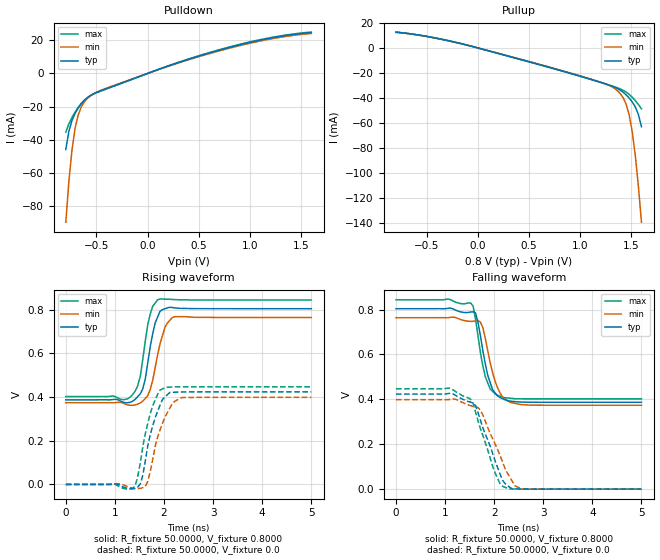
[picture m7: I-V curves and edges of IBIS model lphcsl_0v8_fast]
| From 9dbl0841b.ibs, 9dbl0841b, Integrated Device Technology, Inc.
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|   Model lphcsl_0v8_fast
[Model]  lphcsl_0v8_fast
Model_type Output
Polarity   Non-Inverting
Vmeas =  0.4000V
Cref =   2.0000pF
Rref =   0.0
Vref =   0.4000V
C_comp   1.1000pF   1.0000pF   1.2000pF
[Temperature Range]   27.0000   70.0000   0.0
[Voltage Range]   0.8000V   0.7600V   0.8400V
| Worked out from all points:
|   slope of the pulldown table from 0 to 0.12 V, typ, clamps not added: 44.4 ohm
|   slope of the pullup table from 0 to 0.12 V, typ, clamps not added: 45.4 ohm
|   rising waveform, R_fixture 50.0000, V_fixture 0.8000: 20-80 % time 197ps typ, 236ps min, 183ps max; typ from 0.387 V to 0.804 V
|   rising waveform, R_fixture 50.0000, V_fixture 0.0: 20-80 % time 276ps typ, 307ps min, 256ps max; typ from 0 V to 0.424 V
|   falling waveform, R_fixture 50.0000, V_fixture 0.8000: 20-80 % time 237ps typ, 263ps min, 217ps max; typ from 0.804 V to 0.387 V
|   falling waveform, R_fixture 50.0000, V_fixture 0.0: 20-80 % time 415ps typ, 460ps min, 387ps max; typ from 0.424 V to 0 V
[Pulldown]
|Voltage   I(typ)   I(min)   I(max)
-800mV    -45.83mA   -89.64mA   -35.38mA
-770mV    -34.96mA   -65.18mA   -30.39mA
-740mV    -28.44mA   -46.28mA   -26.61mA
-710mV    -24.18mA   -33.3mA    -23.37mA
-680mV    -20.99mA   -25.25mA   -20.55mA
-650mV    -18.42mA   -20.38mA   -18.13mA
-560mV    -13.36mA   -13.48mA   -13.42mA
-440mV    -10.03mA   -9.766mA   -10.23mA
40mV      915.1uA    880.5uA    940.4uA
610mV     12.43mA    12.04mA    12.7mA
1.15V     20.66mA    20.14mA    20.96mA
1.6V      24.6mA     24.08mA    24.91mA
[Pullup]
|Voltage   I(typ)   I(min)   I(max)
-800mV    12.48mA    12.51mA    12.27mA
-380mV    7.219mA    7.086mA    7.269mA
130mV     -3.031mA   -2.951mA   -3.076mA
1.09V     -24.95mA   -24.74mA   -24.99mA
1.36V     -32.46mA   -34.01mA   -31.91mA
1.42V     -35.56mA   -39.89mA   -34.04mA
1.45V     -37.69mA   -45.23mA   -35.52mA
1.48V     -40.26mA   -53.91mA   -37.39mA
1.51V     -43.39mA   -67.45mA   -39.67mA
1.54V     -47.46mA   -86.58mA   -42.36mA
1.57V     -53.47mA   -111mA     -45.42mA
1.6V      -63.26mA   -139.6mA   -48.89mA
[Ramp]
| variable   typ   min   max
dV/dt_r  0.2541/0.2760n   0.2392/0.3069n   0.2681/0.2545n
dV/dt_f  0.2501/0.2365n   0.2341/0.2632n   0.2651/0.2168n
R_load = 50.0000
[Rising Waveform]
R_fixture= 50.0000
V_fixture= 0.8000
V_fixture_min= 0.7600
V_fixture_max= 0.8400
|time   V(typ)   V(min)   V(max)
0s        387mV      373.7mV    402.1mV
1.31ns    375.8mV    361.9mV    399.5mV
1.46ns    400.6mV    367mV      448.3mV
1.52ns    415.1mV    373mV      497.4mV
1.57ns    439.2mV    381.9mV    576.2mV
1.72ns    630.2mV    435.3mV    779.6mV
1.87ns    765.7mV    592.7mV    844.8mV
2.02ns    803.7mV    718.9mV    847.9mV
2.22ns    807.9mV    767.7mV    845.6mV
5ns       803.9mV    763.8mV    843.9mV
[Rising Waveform]
R_fixture= 50.0000
V_fixture= 0.0
V_fixture_min= 0.0
V_fixture_max= 0.0
|time   V(typ)   V(min)   V(max)
0s        0V         0V         0V
1.41ns    -18.24mV   -18.43mV   -7.708mV
1.52ns    3.168mV    -17.83mV   100.3mV
1.57ns    42.93mV    -14.7mV    174.9mV
1.67ns    177.3mV    14.16mV    280.3mV
1.87ns    334.2mV    216.9mV    412.1mV
2.02ns    399.9mV    308.5mV    442.2mV
2.17ns    421.4mV    370.2mV    445.6mV
2.37ns    423mV      397.7mV    446.6mV
5ns       423.5mV    398.6mV    446.8mV
[Falling Waveform]
R_fixture= 50.0000
V_fixture= 0.8000
V_fixture_min= 0.7600
V_fixture_max= 0.8400
|time   V(typ)   V(min)   V(max)
0s        803.9mV    763.8mV    843.9mV
1.52ns    789.3mV    747.6mV    829.5mV
1.57ns    790.2mV    747.9mV    816.5mV
1.62ns    785mV      749.9mV    757.6mV
1.77ns    615.8mV    719.1mV    547.6mV
1.87ns    506mV      615.7mV    472.2mV
2.07ns    415mV      450.8mV    418.3mV
2.17ns    403.1mV    409.7mV    409.8mV
2.53ns    388.2mV    377.5mV    402.4mV
5ns       387mV      373.7mV    402.1mV
[Falling Waveform]
R_fixture= 50.0000
V_fixture= 0.0
V_fixture_min= 0.0
V_fixture_max= 0.0
|time   V(typ)   V(min)   V(max)
0s        423.5mV    398.6mV    446.8mV
1.06ns    425.8mV    398.7mV    450.5mV
1.52ns    387.9mV    371.7mV    401.1mV
1.62ns    372.3mV    365.8mV    343.4mV
1.72ns    307mV      350.8mV    268.9mV
2.02ns    125.3mV    200.7mV    71.65mV
2.27ns    16.05mV    71.4mV     3.617mV
2.42ns    1.289mV    15.93mV    195.1uV
2.63ns    37.92uV    -294.3uV   -153uV
5ns       657.2nV    0V         711.4nV
